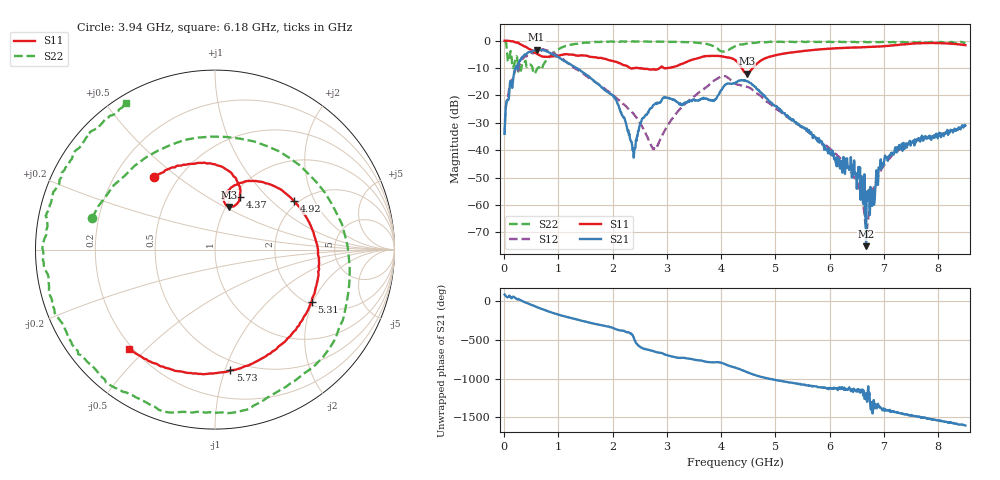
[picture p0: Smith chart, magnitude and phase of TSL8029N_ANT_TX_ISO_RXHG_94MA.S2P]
!Agilent Technologies,E5071C,MY46523237,B.13.01
!Date: Wed Oct 18 10:54:29 2023
!Data & Calibration Information:
!Freq	S11:SOLT2(ON)	S21:SOLT2(ON)	S12:SOLT2(ON)	S22:SOLT2(ON)
!PortZ  Port1:50+j0  Port2:50+j0
!Above PortZ is port z conversion or system Z0 setting when saving the data.
!When reading, reference impedance value at option line is always used.
# Hz S dB R 50
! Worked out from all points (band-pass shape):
!   850 points, 10 MHz to 8.5 GHz, reference 50 ohm
!   highest |S21| = -3.30 dB at 600 MHz (marker M1); lowest = -75.1 dB at 6.67 GHz (marker M2)
!   |S21| within 3 dB of the highest: 320.8 MHz to 1.02 GHz (699.4 MHz wide, 104 % of centre)
!   lowest |S11| = -12.0 dB at 4.47 GHz (marker M3), VSWR 1.67, Z = 51.7 + j26.2 ohm
!   |S11| at or under -10 dB: 2.322 GHz to 2.397 GHz (75.81 MHz wide, 3.21 % of centre); 2.479 GHz to 2.867 GHz (388.8 MHz wide, 14.5 % of centre); 4.38 GHz to 4.58 GHz (199.7 MHz wide, 4.46 % of centre)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
!   |S22| runs from -12.1 to 0.1 dB; largest |S21 - S12| = 0.12
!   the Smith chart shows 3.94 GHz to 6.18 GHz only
!   S11 on the Smith chart (normalised r, x): 3.94 GHz: 0.37, +0.41; 4.37 GHz: 1.08, +0.71; 4.92 GHz: 1.90, +1.40; 5.31 GHz: 2.11, -1.95; 5.73 GHz: 0.42, -1.04; 6.18 GHz: 0.19, -0.44
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1e7  -0.02 -1.9  -34.01 87.9  -34.14 83.5  0.07 -10.4
4e8  -2.25 -74.0  -5.08 -17.9  -5.46 -16.9  -7.48 -155.8
6e8  -4.78 -100.1  -3.30 -73.0  -3.61 -69.6  -10.64 98.7
1.06e9  -5.20 -137.8  -6.84 176.1  -6.35 175.7  -2.47 -96.9
1.43e9  -5.40 171.6  -11.26 108.4  -11.65 112.4  -0.89 -170.2
2.38e9  -10.08 22.6  -39.30 -96.0  -26.62 -4.9  -0.27 67.2
2.84e9  -10.37 -65.4  -22.77 56.2  -37.76 48.9  -0.39 14.1
3.57e9  -6.43 -174.5  -21.94 -41.3  -19.29 -7.5  -0.79 -83.9
3.94e9  -5.56 130.0  -20.01 -66.6  -13.77 -80.6  -3.01 165.5
4.07e9  -5.94 110.2  -16.13 -91.9  -13.00 -119.6  -3.96 77.2
4.26e9  -7.11 79.0  -15.44 -136.1  -15.73 -165.6  -2.03 -22.4
4.37e9  -9.78 64.5  -14.49 -164.3  -16.34 177.4  -1.39 -51.7
4.47e9  -12.03 71.9  -14.76 166.9  -16.81 156.1  -1.05 -72.9
4.92e9  -5.74 31.6  -22.63 74.8  -23.29 77.0  -0.38 -129.4
5.31e9  -4.27 -28.2  -29.10 26.9  -29.22 29.8  -0.39 -165.8
5.67e9  -3.47 -75.5  -34.16 -11.9  -34.36 -9.4  -0.43 163.1
5.73e9  -3.37 -82.7  -35.22 -18.0  -35.25 -16.5  -0.46 158.8
6.18e9  -2.70 -131.1  -45.30 -51.7  -42.70 -60.0  -0.40 121.3
6.67e9  -2.34 -176.7  -75.05 -109.1  -69.74 177.7  -0.52 80.0
7.09e9  -1.90 144.8  -42.08 30.3  -43.28 26.5  -0.51 43.1
7.75e9  -0.88 73.6  -35.01 -60.2  -35.62 -68.7  -0.60 -15.2
8.5e9  -1.64 -19.0  -30.98 -165.1  -30.88 -165.8  -0.99 -89.8
